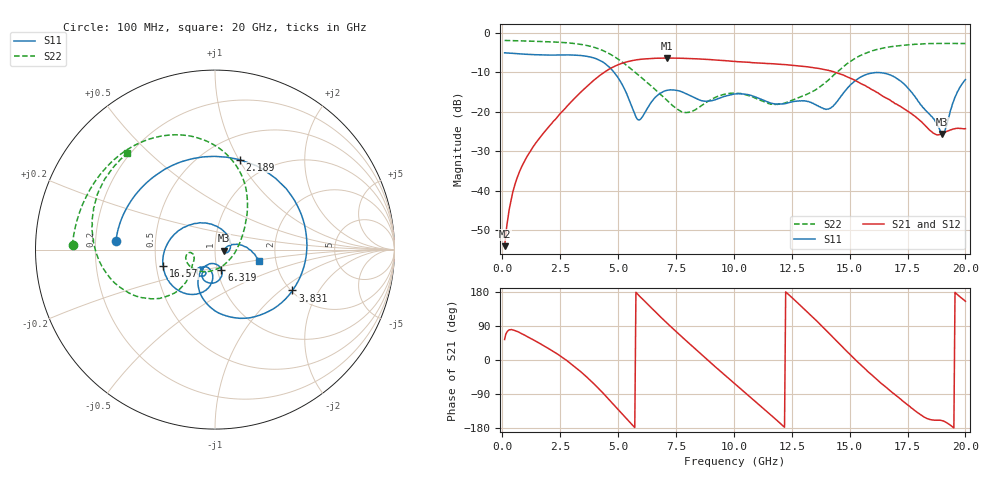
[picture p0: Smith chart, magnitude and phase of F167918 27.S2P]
!  2-Port S-parameters saved by WinCal
! VAR MeasName=S-Parameters (CALIBRATED_DATA) read from VNA (N5242A)
! VAR MeasDate=2016-11-22 10:26:03
! VAR NAME=F167918 27
! VAR FILENAME=F167918 27.S2P
! VAR DATE=2016-11-22 10:26:03
! VAR PHYS_PORTS=1,2
# Hz S DB R 50
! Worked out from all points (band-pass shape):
!   401 points, 100 MHz to 20 GHz, reference 50 ohm
!   highest |S21| = -6.46 dB at 7.115 GHz (marker M1); lowest = -54.0 dB at 100 MHz (marker M2)
!   |S21| within 3 dB of the highest: 4.559 GHz to 14 GHz (9.437 GHz wide, 102 % of centre)
!   lowest |S11| = -25.7 dB at 19 GHz (marker M3), VSWR 1.11, Z = 55.4 - j0.742 ohm
!   |S11| at or under -10 dB: 4.82 GHz to end of sweep
!   |S22| runs from -20.2 to -2.0 dB; largest |S21 - S12| = 0.0029
!   S11 on the Smith chart (normalised r, x): 100 MHz: 0.29, +0.04; 2.189 GHz: 0.73, +1.01; 3.831 GHz: 2.03, -1.21; 6.319 GHz: 1.05, -0.24; 16.57 GHz: 0.54, -0.11; 20 GHz: 1.63, -0.23
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1e8  -5.13 175.1  -53.99 54.1  -53.74 55.0  -2.00 178.3
7.4675e8  -5.39 145.0  -35.11 72.3  -35.05 72.0  -2.10 167.9
2.1895e9  -5.69 74.7  -22.55 23.0  -22.56 22.8  -2.37 143.8
3.43325e9  -5.83 -0.7  -14.82 -33.3  -14.83 -33.2  -3.03 117.1
3.83125e9  -6.23 -27.8  -12.68 -55.4  -12.67 -55.3  -3.51 106.7
4.92575e9  -10.80 -102.3  -8.33 -125.5  -8.31 -125.7  -6.41 75.3
5.82125e9  -21.84 -106.3  -6.87 175.2  -6.87 175.1  -10.45 53.0
6.31875e9  -18.65 -72.2  -6.59 144.3  -6.58 144.3  -12.95 41.0
6.7665e9  -15.58 -80.5  -6.48 117.5  -6.48 117.5  -15.29 27.3
7.11475e9  -14.59 -92.3  -6.46 97.3  -6.46 97.4  -17.15 13.0
8.60725e9  -17.23 -116.8  -6.70 14.1  -6.69 14.1  -18.44 -98.3
1.005e10  -15.52 -117.9  -7.29 -63.1  -7.28 -63.0  -15.33 -158.5
1.089575e10  -16.20 -130.3  -7.64 -107.4  -7.60 -107.5  -16.50 -172.9
1.189075e10  -18.07 -126.0  -7.99 -161.1  -7.96 -161.1  -18.16 -161.6
1.338325e10  -17.84 -126.8  -8.82 114.4  -8.79 114.6  -14.97 -138.9
1.407975e10  -19.37 -110.8  -9.54 72.6  -9.53 72.5  -12.04 -131.7
1.4826e10  -14.61 -95.8  -11.03 26.0  -10.96 26.3  -8.16 -137.0
1.656725e10  -10.35 -162.8  -16.53 -71.6  -16.42 -71.7  -3.79 -174.1
1.67165e10  -10.66 -170.8  -16.95 -79.4  -16.98 -79.3  -3.65 -177.0
1.77115e10  -15.31 119.2  -20.68 -128.3  -20.61 -128.3  -3.02 165.1
1.9005e10  -25.66 -7.4  -25.55 -160.4  -25.45 -160.0  -2.75 145.2
2e10  -11.90 -15.1  -24.30 155.1  -24.16 155.6  -2.77 132.3
